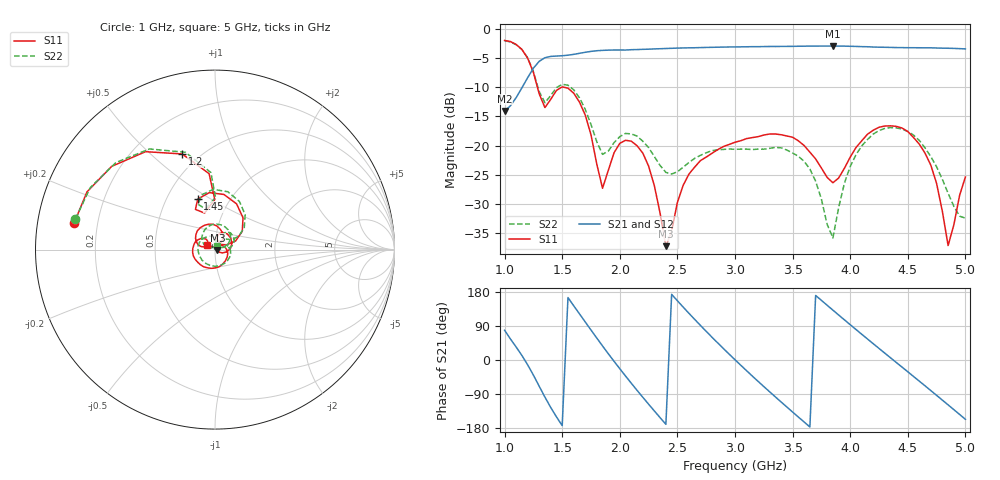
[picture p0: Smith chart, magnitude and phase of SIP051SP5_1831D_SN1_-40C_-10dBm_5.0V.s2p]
# GHz  S  dB  R  50
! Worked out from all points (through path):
!   81 points, 1 GHz to 5 GHz, reference 50 ohm
!   highest |S21| = -2.90 dB at 3.85 GHz (marker M1); lowest = -14.1 dB at 1 GHz (marker M2)
!   lowest |S11| = -37.3 dB at 2.4 GHz (marker M3), VSWR 1.03, Z = 51.4 - j0.202 ohm
!   |S11| at or under -10 dB: 1.285 GHz to 1.494 GHz (208.5 MHz wide, 15 % of centre); 1.518 GHz to end of sweep
!   |S22| runs from -35.9 to -2.0 dB; largest |S21 - S12| = 0.0021
!   S11 on the Smith chart (normalised r, x): 1 GHz: 0.11, +0.09; 1.2 GHz: 0.41, +0.63; 1.45 GHz: 0.71, +0.44; 5 GHz: 0.91, +0.05
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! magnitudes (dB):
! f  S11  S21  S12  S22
! 1 GHz  -1.9  -14.1  -14.1  -2.0
! 1.2 GHz  -5.0  -8.3  -8.3  -4.9
! 1.35 GHz  -13.5  -4.9  -4.9  -12.7
! 1.45 GHz  -10.5  -4.6  -4.6  -10.1
! 1.7 GHz  -14.8  -4.0  -4.0  -13.8
! 1.85 GHz  -27.3  -3.6  -3.6  -21.5
! 2 GHz  -19.6  -3.6  -3.6  -18.5
! 2.1 GHz  -19.3  -3.5  -3.5  -18.0
! 2.25 GHz  -23.5  -3.4  -3.4  -20.4
! 2.35 GHz  -31.7  -3.4  -3.4  -23.4
! 2.4 GHz  -37.3  -3.3  -3.3  -24.6
! 2.6 GHz  -24.9  -3.2  -3.2  -22.9
! 3 GHz  -19.4  -3.1  -3.1  -20.7
! 3.45 GHz  -18.4  -3.0  -3.0  -20.8
! 3.7 GHz  -22.3  -2.9  -2.9  -26.1
! 3.85 GHz  -26.4  -2.9  -2.9  -35.9
! 4.05 GHz  -20.3  -3.0  -3.0  -21.6
! 4.35 GHz  -16.6  -3.1  -3.1  -16.9
! 4.65 GHz  -21.3  -3.2  -3.2  -20.4
! 4.75 GHz  -26.5  -3.2  -3.2  -23.7
! 4.85 GHz  -37.2  -3.3  -3.3  -28.2
! 5 GHz  -25.4  -3.4  -3.4  -32.5
